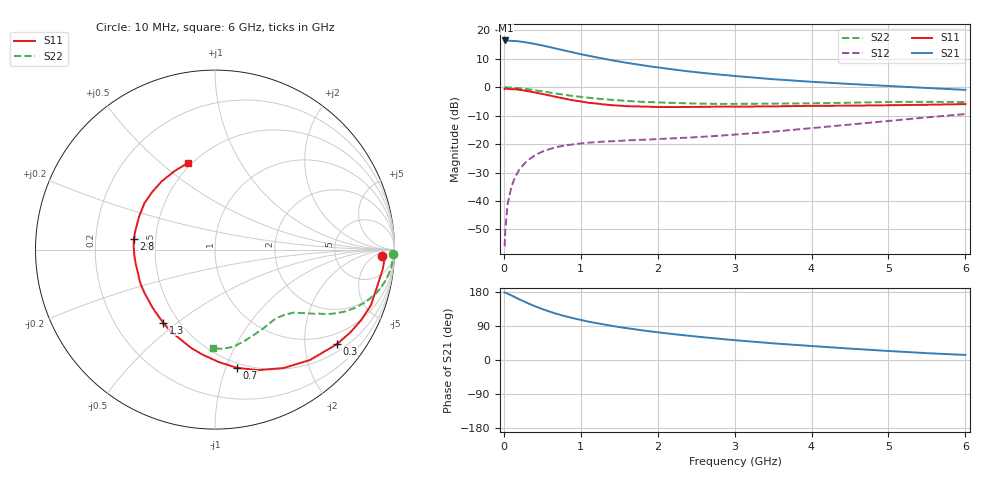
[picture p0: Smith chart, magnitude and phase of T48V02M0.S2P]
! Infineon Technologies  Discrete & RF Semiconductors
! BFR182T
! Si NPN RF Bipolar Junction Transistor in SC75
! VCE = 8 V  IC = 2 mA
! Common Emitter S-Parameters:  October  1999
# GHz  S  MA  R  50
!  f  S11  S21  S12  S22
! GHz  MAG  ANG  MAG  ANG  MAG  ANG  MAG  ANG
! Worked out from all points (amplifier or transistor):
!   36 points, 10 MHz to 6 GHz, reference 50 ohm
!   highest |S21| = 16.5 dB at 20 MHz (marker M1)
!   |S21| within 3 dB of that: start of sweep to 702 MHz
!   unconditionally stable (mu >= 1): 2.077 GHz to 4.413 GHz
!   at 250 MHz: K = 0.14, MSG = 21.7 dB, |S12| = -27.4 dB
!   at 1.4 GHz: K = 0.76, MSG = 14.3 dB, |S12| = -19.0 dB
!   at 6 GHz: K = 0.83, MSG = 4.3 dB, |S12| = -9.4 dB
!   lowest NFmin = 1.10 dB at 450 MHz
!   S11 on the Smith chart (normalised r, x): 10 MHz: 21, -12; 300 MHz: 0.69, -2.76; 700 MHz: 0.46, -1.09; 1.3 GHz: 0.41, -0.45; 2.8 GHz: 0.38, +0.05; 6 GHz: 0.48, +0.62
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0.01  0.9297 -2.3  6.603 178.2  0.0016 83.8  0.9894 -1.3
0.02  0.9498 -1.4  6.665 178.1  0.0033 95.9  0.9999 -1.1
0.05  0.9411 -6.6  6.623 175.0  0.0089 90.3  0.9924 -2.8
0.1  0.927 -12.5  6.554 170.4  0.0181 83.1  0.9879 -5.5
0.15  0.9226 -19.6  6.509 165.2  0.0269 79.0  0.9764 -8.1
0.2  0.9041 -25.8  6.418 160.3  0.0354 76.5  0.9636 -10.6
0.3  0.859 -37.9  6.127 151.0  0.0504 69.5  0.9304 -15.2
0.4  0.8115 -49.3  5.801 142.2  0.0632 63.7  0.8893 -19.2
0.5  0.7627 -59.9  5.437 134.5  0.0737 58.7  0.8475 -22.4
0.6  0.7138 -70.2  5.074 127.3  0.0821 54.7  0.8067 -25.2
0.7  0.6695 -79.6  4.725 121.1  0.0896 51.5  0.7684 -27.4
0.9  0.5895 -96.7  4.101 110.3  0.0988 46.6  0.7021 -30.7
1.1  0.5337 -111.7  3.594 101.2  0.1061 43.6  0.6546 -33.1
1.3  0.499 -125.4  3.187 93.8  0.1109 42.0  0.6154 -35.1
1.6  0.465 -143.2  2.688 83.9  0.1162 41.1  0.575 -37.6
1.9  0.4546 -157.5  2.331 75.6  0.1206 42.1  0.5484 -40.5
2.2  0.4487 -169.0  2.062 68.4  0.1263 43.9  0.5311 -43.3
2.8  0.4557 172.8  1.674 56.1  0.1403 48.7  0.5107 -50.2
3.5  0.4615 156.3  1.386 44.0  0.1657 54.2  0.5148 -58.7
4.5  0.4748 137.5  1.143 30.1  0.2209 57.9  0.5351 -72.2
5.5  0.4923 117.1  0.973 18.0  0.2952 56.7  0.5545 -85.5
6  0.5057 107.4  0.901 13.4  0.338 54.2  0.5506 -91.4
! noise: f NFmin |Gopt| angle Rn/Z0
0.45  1.1  0.42  29  0.36
0.9  1.2  0.4  58  0.3
1.8  1.85  0.32  126  0.22
